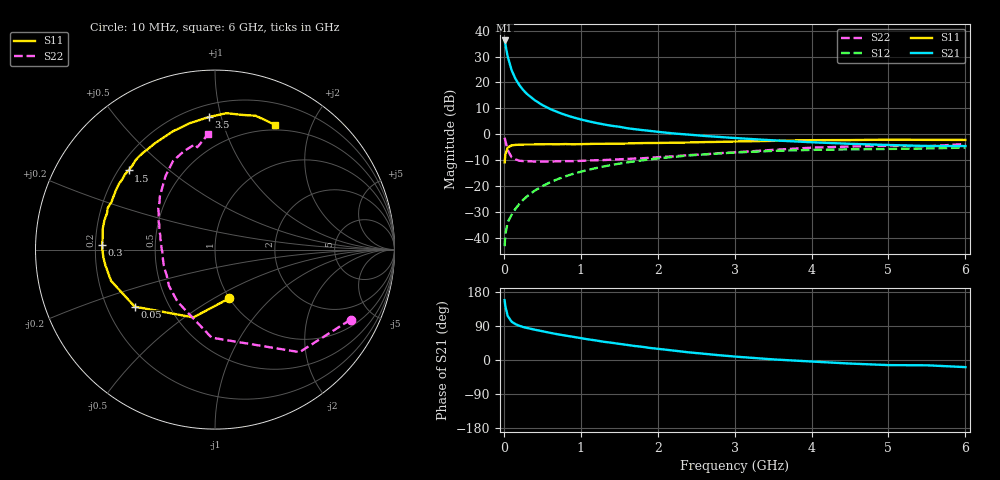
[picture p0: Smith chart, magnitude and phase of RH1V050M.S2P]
! SIEMENS Small Signal Semiconductors
! BFR106
! Si NPN RF Bipolar Junction Transistor in SOT23
! VCE = 1 V  IC = 50 mA
! Common Emitter S-Parameters:  August  1996
# GHz  S  MA  R  50
!  f  S11  S21  S12  S22
! GHz  MAG  ANG  MAG  ANG  MAG  ANG  MAG  ANG
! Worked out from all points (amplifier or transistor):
!   36 points, 10 MHz to 6 GHz, reference 50 ohm
!   highest |S21| = 36.2 dB at 10 MHz (marker M1)
!   |S21| within 3 dB of that: start of sweep to 29.48 MHz
!   unconditionally stable (mu >= 1): 199.6 MHz to end of sweep
!   at 250 MHz: K = 1.04, MAG = 20.0 dB, |S12| = -25.4 dB
!   at 1.4 GHz: K = 1.08, MAG = 5.9 dB, |S12| = -12.0 dB
!   at 6 GHz: K = 1.02, MAG = -0.7 dB, |S12| = -5.2 dB
!   S11 on the Smith chart (normalised r, x): 10 MHz: 1.00, -0.59; 50 MHz: 0.32, -0.29; 300 MHz: 0.23, +0.02; 1.5 GHz: 0.24, +0.37; 3.5 GHz: 0.28, +0.92; 6 GHz: 0.44, +1.50
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0.01  0.283 -73.8  64.61 157.9  0.0068 74.6  0.8503 -27.3
0.02  0.3965 -107.7  54.28 141.4  0.0116 62.6  0.7405 -50.5
0.05  0.5488 -144.6  31.57 116.2  0.0197 54.6  0.491 -92.2
0.1  0.6049 -163.3  17.36 101.4  0.0274 57.8  0.358 -125.6
0.15  0.6168 -171.8  11.8 94.7  0.0358 61.8  0.3262 -142.0
0.2  0.6236 -176.1  8.945 90.4  0.0443 64.9  0.3056 -151.4
0.25  0.6269 -179.6  7.147 87.1  0.0534 66.7  0.3005 -158.8
0.3  0.6289 177.6  5.989 84.6  0.0622 68.3  0.2986 -162.9
0.4  0.6301 173.2  4.537 80.1  0.0803 69.2  0.295 -169.7
0.5  0.6363 169.3  3.65 76.0  0.0983 69.0  0.2934 -174.5
0.6  0.6374 165.1  3.066 71.8  0.1165 68.3  0.2938 -177.8
0.7  0.635 161.3  2.659 67.9  0.1344 67.3  0.2973 179.4
0.8  0.6412 158.8  2.342 64.5  0.1526 65.6  0.2996 176.3
1.1  0.6439 148.8  1.768 54.4  0.2039 60.9  0.3087 169.7
1.5  0.6532 137.5  1.385 42.6  0.2678 53.8  0.3251 161.7
1.7  0.6658 131.8  1.243 37.0  0.2965 50.0  0.3363 157.4
2.2  0.6806 119.4  1.031 25.0  0.3621 40.9  0.3704 147.8
2.8  0.7066 105.4  0.881 12.6  0.4225 30.3  0.4272 136.0
3.5  0.7395 92.6  0.757 1.6  0.4729 19.3  0.4947 123.8
4.5  0.7655 78.7  0.649 -9.4  0.5059 5.5  0.5745 107.7
5.5  0.7731 68.0  0.589 -14.0  0.5265 -2.5  0.579 99.8
6  0.7706 64.2  0.587 -18.8  0.5489 -8.9  0.6426 93.5
